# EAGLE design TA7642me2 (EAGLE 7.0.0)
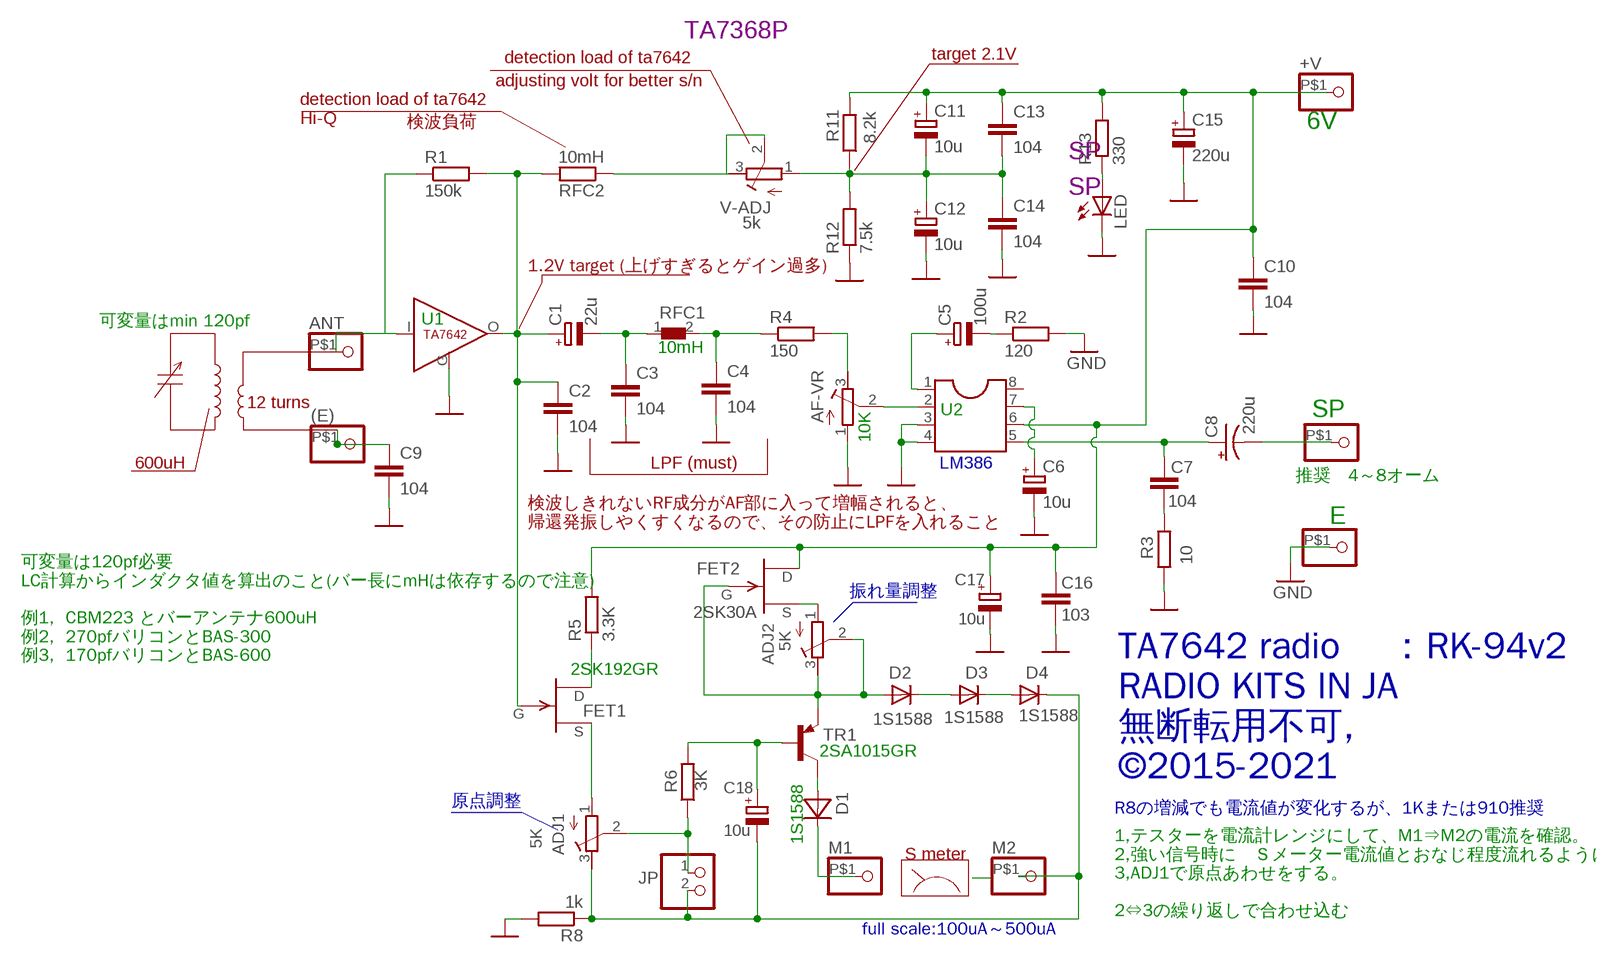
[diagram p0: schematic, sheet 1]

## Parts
(E)  PINHD-1X1  [1X01]
+V  PINHD-1X1  [1X01]
ADJ1  5K  R-TRIMM3296W  [RTRIM3296W]
ADJ2  5K  R-TRIMM3296W  [RTRIM3296W]
AF-VR  20K  R-TRIMM3296W  [RTRIM3296W]
ANT  PINHD-1X1  [1X01]
C1  22u  CPOL-EUE2.5-5  [E2,5-5]
C2  104  C-EU050-024X044  [C050-024X044]
C3  104  C-EU050-024X044  [C050-024X044]
C4  104  C-EU050-024X044  [C050-024X044]
C5  100u  CPOL-EUE2.5-7  [E2,5-7]
C6  10u  CPOL-EUE2.5-6  [E2,5-6]
C7  104  C-EU050-024X044  [C050-024X044]
C8  220u  CPOL-USE2.5-7  [E2,5-7]
C9  104  C-EU050-024X044  [C050-024X044]
C10  104  C-EU050-024X044  [C050-024X044]
C11  10u  CPOL-EUE2.5-6  [E2,5-6]
C12  10u  CPOL-EUE2.5-6  [E2,5-6]
C13  104  C-EU050-024X044  [C050-024X044]
C14  104  C-EU050-024X044  [C050-024X044]
C15  220u  CPOL-EUE2.5-7  [E2,5-7]
C16  103  C-EU050-024X044  [C050-024X044]
C17  10u  CPOL-EUE2.5-5  [E2,5-5]
C18  10u  CPOL-EUE2.5-5  [E2,5-5]
D1  1N60  [DO34-5]
D2  1S1588  DIODE-D-5  [D-5]
D3  1S1588  DIODE-D-5  [D-5]
D4  1S1588  DIODE-D-5  [D-5]
E  PINHD-1X1  [1X01]
FET1  2SK192A  [2SK192A]
FET2  2SK30A  [2SK30]
JP  PINHD-1X2  [1X02]
LED  LEDIRL80A  [IRL80A]
M1  PINHD-1X1  [1X01]
M2  PINHD-1X1  [1X01]
R1  150k  R-EU_0204/5  [0204/5]
R2  120  R-EU_0204/5  [0204/5]
R3  10  R-EU_0204/5  [0204/5]
R4  150  R-EU_0204/5  [0204/5]
R5  3.3K  R-EU_0204/5  [0204/5]
R6  3K  R-EU_0204/5  [0204/5]
R8  1k  R-EU_0204/5  [0204/5]
R11  8.2k  R-EU_0204/5  [0204/5]
R12  7.5k  R-EU_0204/5  [0204/5]
R13  330  R-EU_0204/5  [0204/5]
RFC1  8101  [8101]
RFC2  10mH  R-EU_0204/7  [0204/7]
SP  PINHD-1X1  [1X01]
TR1  2SA1015  [TO92-BCE]
U1  TA7642  [TA7642]
U2  LM386  [DIL08]
V-ADJ  5k  R-TRIMM3296W  [RTRIM3296W]

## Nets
5V1: +V.P$1 C10.1 C11.+ C13.1 C15.+ C16.1 C17.+ FET2.D R5.2 R11.2 R13.2 U2.6
GND: AF-VR.1(E) C2.2 C3.2 C4.2 C6.- C9.2 C10.2 C12.- C14.2 C15.- C16.2 C17.- E.P$1 LED.K(C) R2.2 R3.2 R8.2 R12.1 U1.G(GND) U2.3 U2.4
N$1: ANT.P$1 R1.1 U1.I(IN)
N$2: C1.+ C2.1 FET1.G R1.2 RFC2.2 U1.O(OUT)
N$3: RFC2.1 V-ADJ.2(S) V-ADJ.3(A)
N$4: C11.- C12.+ C13.2 C14.1 R11.1 R12.2 V-ADJ.1(E)
N$5: (E).P$1 C9.1
N$6: LED.A R13.1
N$7: C1.- C3.1 RFC1.1
N$8: AF-VR.3(A) R4.2
N$9: ADJ1.1(E) FET1.S
N$11: ADJ2.1(E) FET2.S
N$12: C4.1 R4.1 RFC1.2
N$13: C5.+ U2.1
N$14: C5.- R2.1
N$15: C7.1 R3.1
N$16: AF-VR.2(S) U2.2
N$17: ADJ2.2(S) ADJ2.3(A) D2.A FET2.G TR1.E
N$18: ADJ1.3(A) C18.- D4.C JP.2 M2.P$1 R8.1
N$19: C18.+ R6.2 TR1.B
N$20: D1.A TR1.C
N$21: D1.C M1.P$1
N$22: ADJ1.2(S) JP.1 R6.1
N$23: D2.C D3.A
N$24: FET1.D R5.1
N$25: D3.C D4.A
N$29: C6.+ U2.7
N$33: C8.- SP.P$1
N$34: C7.2 C8.+ U2.5
Unconnected: U2.8

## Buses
B$1
B$2

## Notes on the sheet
- TA7368P
- detection load of ta7642 | target 2.1V
- adjusting volt for better s/n
- detection load of ta7642
  Hi-Q
- 検波負荷 | 6V
- SP
- SP
- 1.2V target (上げすぎるとゲイン過多)
- 可変量はmin 120pf | U1
- 10mH
- 12 turns
- U2 | SP
- 10K
- 600uH | LPF (must)
- 推奨　4～8オーム
- E
- 検波しきれないRF成分がAF部に入って増幅されると、
  帰還発振しやくすくなるので、その防止にLPFを入れること
- 振れ量調整
- 可変量は120pf必要
  LC計算からインダクタ値を算出のこと(バー長にmHは依存するので注意)
  
  例1,  CBM223 とバーアンテナ600uH
  例2,  270pfバリコンとBAS-300　
  例3,  170pfバリコンとBAS-600
- 2SK192GR
- 2SA1015GR
- TA7642 radio 　：RK-94v2
  RADIO KITS IN JA
  無断転用不可, 
  ©2015-2021
- 原点調整
- R8の増減でも電流値が変化するが、1Kまたは910推奨
- 1S1588
- S meter
- full scale:100uA～500uA
- 1,テスターを電流計レンジにして、M1⇒M2の電流を確認。
  2,強い信号時に　Ｓメーター電流値とおなじ程度流れるようにADJ2を合わせる。
  3,ADJ1で原点あわせをする。
  
  2⇔3の繰り返しで合わせ込む

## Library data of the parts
(E) +V ANT E M1 M2 SP = pinhead:PINHD-1X1: PIN HEADER
ADJ1 ADJ2 AF-VR V-ADJ = resistor:R-TRIMM: Trimm resistor
C1 C5 C6 C11 C12 C15 C17 C18 = resistor:CPOL-EU: POLARIZED CAPACITOR, European symbol
C2-C4 C7 C9 C10 C13 C14 C16 = resistor:C-EU: CAPACITOR, European symbol
C8 = resistor:CPOL-US: POLARIZED CAPACITOR, American symbol
D1 = diode:1N60
D2-D4 = diode:DIODE-: DIODE
FET1 = transistor-fet:2SK192A
FET2 = transistor-fet:2SK30A
JP = pinhead:PINHD-1X2: PIN HEADER
LED = led:LED: LED
R1-R6 R8 R11-R13 RFC2 = resistor:R-EU_: RESISTOR, European symbol
RFC1 = inductors:8101
TR1 = transistor-pnp:2SA1015
U1 = AN217:TA7642
U2 = ic-package:LM386

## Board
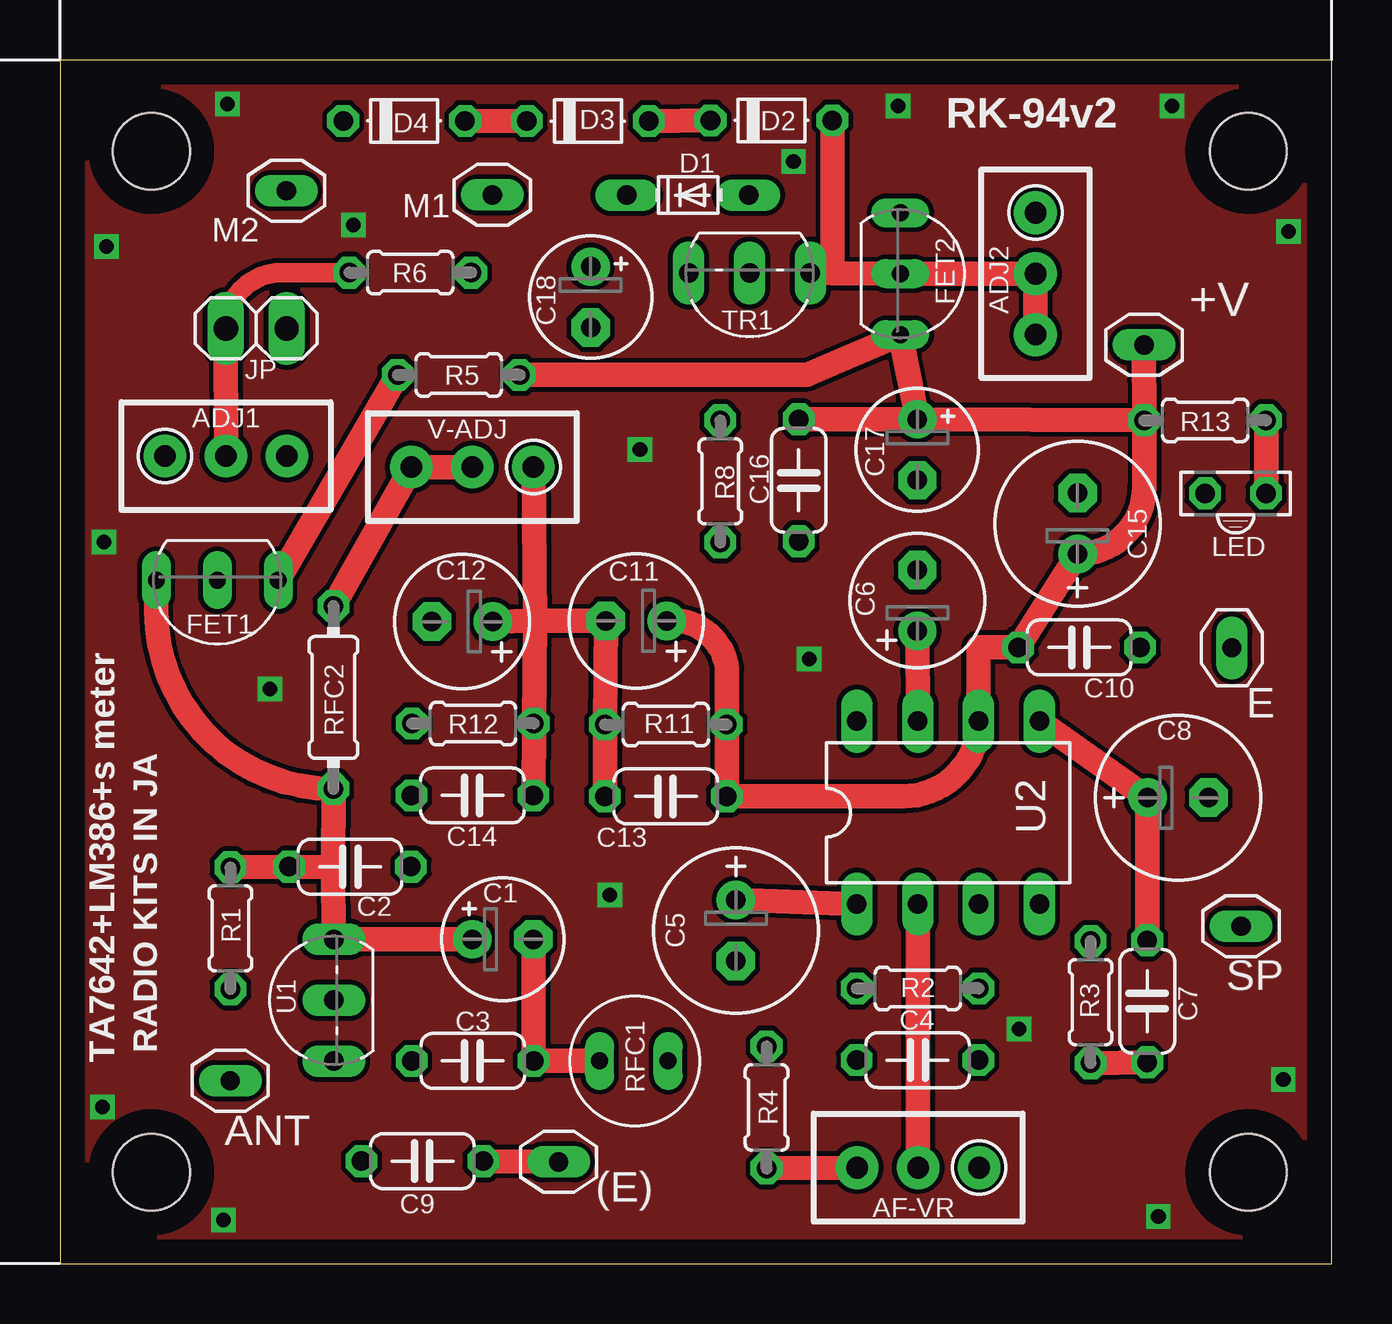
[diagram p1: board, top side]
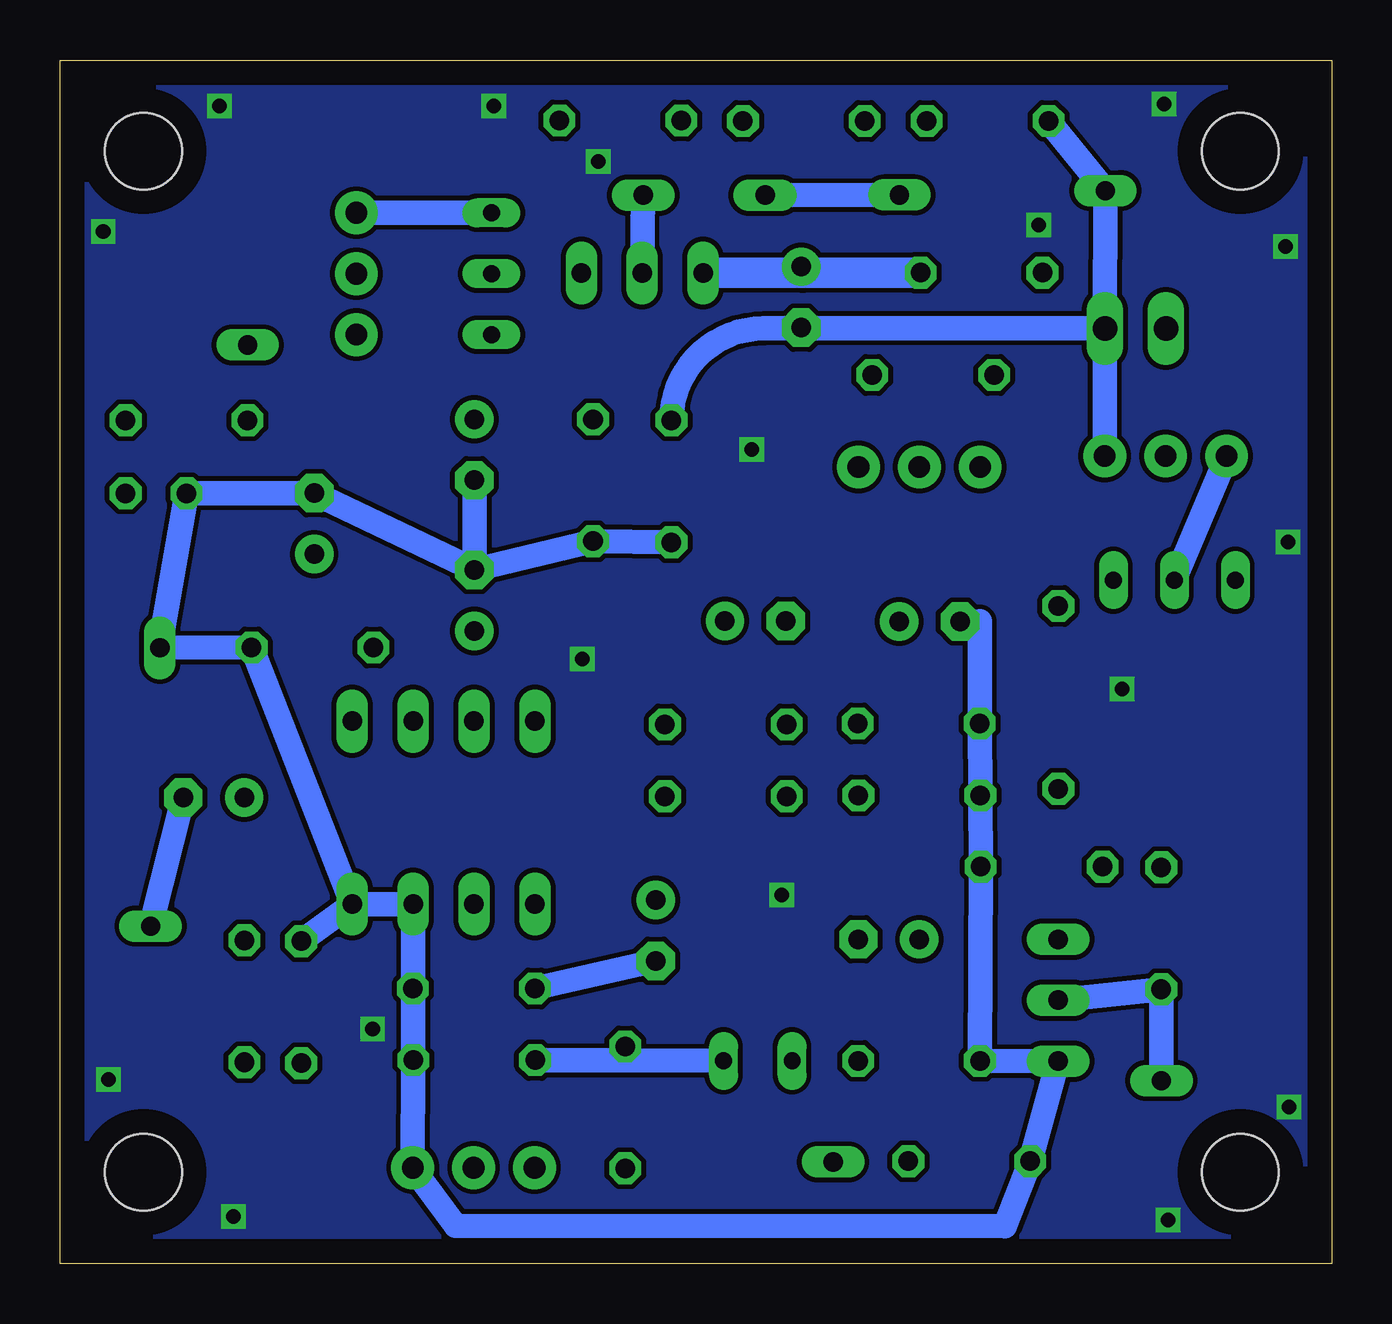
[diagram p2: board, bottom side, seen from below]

Size 53.01 x 50.16 mm. Coordinates in mm from the lower left corner, seen from the top.
Outline: 0,0 53.01,0 53.01,50.16 0,50.16 0,0
Copper layers (1*16): Top 0.035mm / dielectric 1.5mm / Bottom 0.035mm
Design rules "default": minimum track width 10mil, minimum drill 24mil, track to track 8mil, track to pad 8mil, pad to pad 8mil, via to via 8mil, smd to smd 8mil, copper to edge 40mil, drill to drill 8mil, minimum pad ring 10mil, minimum via ring 8mil, stop-mask expansion 4mil, vias tented up to drill 0mil, thermal gap 10mil
Holes 3.2 mm at 3.81,3.81 49.53,3.81 3.81,46.35 49.53,46.35

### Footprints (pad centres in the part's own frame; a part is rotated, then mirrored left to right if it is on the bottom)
1X01 = drill 0.8 long: P$1 0,0
RTRIM3296W = drill 0.9 pad 1.778: 1 0,-2.54; 2 0,0; 3 0,2.54
E2,5-5 = drill 0.813 pad 1.6: + -1.27,0 | drill 0.813 pad 1.6 octagon: - 1.27,0
C050-024X044 = drill 0.813 octagon: 1 -2.54,0; 2 2.54,0
E2,5-7 = drill 0.813 pad 1.6: + -1.27,0 | drill 0.813 pad 1.6 octagon: - 1.27,0
E2,5-6 = drill 0.813 pad 1.6: + -1.27,0 | drill 0.813 pad 1.6 octagon: - 1.27,0
DO34-5 = drill 0.813 long: A 2.54,0; C -2.54,0
D-5 = drill 0.813 octagon: A 2.54,0; C -2.54,0
2SK192A = drill 0.7 pad 1.016 long: D -3.81,0; G 1.27,0; S -1.27,0
2SK30 = drill 0.7 pad 1.016 long: D 2.54,0; G 0,0; S -2.54,0
1X02 = drill 1.016 long: 1 -1.27,0; 2 1.27,0
IRL80A = drill 0.813 octagon: A 0,-1.27; K 0,1.27
0204/5 = drill 0.813 octagon: 1 -2.54,0; 2 2.54,0
8101 = drill 0.7 pad 0.813 long: 1 0,1.46; 2 0,-1.397
0204/7 = drill 0.813 octagon: 1 -3.81,0; 2 3.81,0
TO92-BCE = drill 0.813 long: B 2.54,0; C 0,0; E -2.54,0
TA7642 = drill 0.813 long: G -2.54,0; I 0,0; O 2.54,0
DIL08 = drill 0.813 long: 1 -3.81,-3.81; 2 -1.27,-3.81; 3 1.27,-3.81; 4 3.81,-3.81; 5 3.81,3.81; 6 1.27,3.81; 7 -1.27,3.81; 8 -3.81,3.81

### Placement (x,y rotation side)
(E)  20.78,4.24 180 top
+V  45.19,38.28 180 top
ADJ1  6.92,33.66 270 top
ADJ2  40.66,41.25 180 top
AF-VR  35.77,4 90 top
ANT  7.1,7.63 0 top
C1  18.46,13.52 0 top
C2  12.09,16.54 0 top
C3  17.2,8.45 180 top
C4  35.74,8.48 0 top
C5  28.17,13.89 270 top
C6  35.74,27.64 90 top
C7  45.32,10.93 90 top
C8  46.6,19.42 0 top
C9  15.11,4.27 180 top
C10  42.48,25.68 0 top
C11  24.02,26.78 180 top
C12  16.76,26.76 180 top
C13  25.25,19.48 180 top
C14  17.19,19.51 180 top
C15  42.41,30.84 90 top
C16  30.79,32.65 270 top
C17  35.74,33.92 270 top
C18  22.12,40.27 270 top
D1  26.16,44.53 0 top
D2  29.65,47.64 0 top
D3  22,47.61 0 top
D4  14.34,47.62 0 top
E  48.84,25.66 90 top
FET1  5.29,28.48 180 top
FET2  35.03,41.25 270 top
JP  8.18,38.97 0 top
LED  49,32.1 90 top
M1  18.02,44.53 0 top
M2  9.44,44.71 180 top
R1  7.11,13.98 90 top
R2  35.76,11.47 0 top
R3  42.96,10.9 90 top
R4  29.45,6.52 270 top
R5  16.62,37.03 0 top
R6  14.6,41.29 0 top
R8  27.52,32.6 270 top
R11  25.25,22.47 0 top
R12  17.21,22.51 0 top
R13  47.73,35.14 180 top
RFC1  23.95,8.45 90 top
RFC2  11.4,23.6 270 top
SP  49.23,14.07 0 top
TR1  28.74,41.28 180 top
U1  11.41,10.98 90 top
U2  37.02,18.8 0 top
V-ADJ  17.19,33.19 90 top

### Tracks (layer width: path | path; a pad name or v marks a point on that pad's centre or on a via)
5V1
  Top 1.016: C11.+ arc-90 27.81,24.77 R11.2 C13.1 35.16,19.48 arc90 U2.6 38.28,25.68 C10.1 C15.+ arc90 45.19,32.35 R13.2 | +V.P$1 R13.2 | R5.2 31.14,37.05 FET2.D C17.+ | R13.2 C17.+ | C16.1 C17.+
GND
  Bottom 0.254: 14.68,26.77 C12.-
  Bottom 1.016: U2.4 U2.3 R2.2 C4.2 AF-VR.1 36.51,1.59 13.63,1.57 C9.2 U1.G C3.2 C2.2 C14.2 R12.1 14.68,26.77 | R3.2 U2.4 | U2.4 C10.2 E.P$1 LED.K C15.- C6.- | C6.- C16.2 R8.2 | C17.- C6.-
GND2  (via drill 0.61)
  other vias: 1.93,42.39 46.36,48.24 45.78,1.97 22.92,15.37 50.99,7.68 6.82,1.83 39.98,9.77 51.21,43.01 1.78,6.53 31.24,25.2 1.83,30.07 6.99,48.32 30.58,45.93 12.22,43.28 8.74,23.94 24.17,33.93 34.93,48.24
  pour Top: -0.88,52.01 54.36,52.01 55.24,-1.27 0,-1.27
  pour Bottom: -0.66,51.22 53.34,52.7 53.98,-1.27 0,-1.27
N$1
  Bottom 1.016: ANT.P$1 R1.1 U1.I
N$2
  Top 1.016: C1.+ U1.O 11.38,16.53 | R1.2 C2.1 11.38,16.53 | 11.38,16.53 RFC2.2 arc-90 4.02,27.16 FET1.G
N$3
  Top 1.016: RFC2.1 V-ADJ.3 V-ADJ.2
N$4
  Top 1.016: C13.2 R11.1 C11.- 19.79,26.78 | C14.1 R12.2 19.79,26.78 | V-ADJ.1 19.79,26.78 | C12.+ 19.79,26.78
N$5
  Top 1.016: (E).P$1 C9.1
N$6
  Top 1.016: R13.1 LED.A
N$7
  Top 1.016: RFC1.1 C3.1 C1.-
N$8
  Top 1.016: AF-VR.3 R4.2
N$9
  Bottom 1.016: ADJ1.1 FET1.S
N$11
  Bottom 1.016: FET2.S ADJ2.1
N$12
  Bottom 1.016: C4.1 29.21,8.47 | 29.21,8.47 RFC1.2 | R4.1 29.21,8.47
N$13
  Top 1.016: U2.1 C5.+
N$14
  Bottom 1.016: R2.1 C5.-
N$15
  Top 1.016: C7.1 R3.1
N$16
  Top 1.016: U2.2 AF-VR.2
N$17
  Top 1.016: TR1.E 32.19,41.27 | 32.19,41.27 FET2.G ADJ2.2 ADJ2.3 | D2.A 32.19,41.27
N$18
  Bottom 0.254: C18.- 22.18,39 22.18,38.97
  Bottom 1.016: ADJ1.3 JP.2 | JP.2 M2.P$1 D4.C | JP.2 22.18,38.97 23.69,38.97 arc-90 R8.1
N$19
  Bottom 0.254: C18.+ 22.06,41.54 22.06,41.29
  Bottom 1.27: R6.2 22.06,41.29 TR1.B
N$20
  Bottom 1.016: TR1.C D1.A
N$21
  Bottom 1.016: D1.C M1.P$1
N$22
  Top 0.813: R6.1 9.23,41.29 arc90 JP.1
  Top 1.016: JP.1 ADJ1.2
N$23
  Top 1.016: D3.A D2.C
N$24
  Top 1.016: R5.1 FET1.D
N$25
  Top 1.016: D3.C D4.A
N$29
  Top 1.016: U2.7 C6.+
N$33
  Bottom 1.016: C8.- SP.P$1
N$34
  Top 1.016: U2.5 C8.+ C7.2

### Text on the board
tNames: RK-94v2 | RADIO KITS IN JA | TA7642+LM386+s meter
